FUNCTION_BLOCK FB_FileCopy
(*SwenChen 2011.4.13 ÐÞ¸ÄÓÚ°ïÖúÎÄ¼þ*)
VAR_INPUT
	srcNetId				: T_AmsNetId;	(* TwinCAT network address of the source file *)
	srcFileName			: T_MaxString;	(* source file path and name *)
	destNetId			: T_AmsNetId;	(* TwinCAT network address of the destination file *)
	destFileName		: T_MaxString;  (* destination file path and name *)
	bExecute			: BOOL;			(* rising edge start fb execution *)
	tAdsTimeOut			: TIME;			(* ads timeout *)
	cbReadLen			: UDINT;
END_VAR
VAR_OUTPUT
	bBusy				:BOOL;
	bError				:BOOL;
	nErrId				:UDINT;
END_VAR
VAR
	fbFileOpen			:FB_FileOpen;
	fbFileClose			:FB_FileClose;
	fbFileRead			:FB_FileRead;
	fbFileWrite			:FB_FileWrite;

	hSrcFile				:UINT	:= 0;(* file handle of the source file *)
	hDestFile			:UINT	:= 0;(* file handle of the destination file *)

	Step				:DWORD;
	RisingEdge			:R_TRIG;

	buffRead				:ARRAY[1..30000] OF BYTE;(* buffer *)
	cbReadLength		:UDINT:=0;
	TimeCount			:INT;
END_VAR

RisingEdge(CLK:=bExecute);
IF RisingEdge.Q THEN
	IF NOT bBusy THEN
		bBusy := TRUE;
		bError:= FALSE;
		nErrId:=0;
		Step := 1;
		cbReadLength:=0;
		hSrcFile:=0;
		hDestFile:=0;
		TimeCount:=0;
	END_IF
END_IF

IF bBusy THEN
	TimeCount:=TimeCount+1;
END_IF


CASE Step OF
	0:	(* do nothing *)
		;

	1:	(* open source file *)
		fbFileOpen(  bExecute := FALSE  );
		fbFileOpen( 	sNetId := srcNetId,
						sPathName := srcFileName,
						nMode := FOPEN_MODEREAD OR FOPEN_MODEBINARY(*FOPEN_MODETEXT*),
						ePath := PATH_GENERIC,
						tTimeout := tAdsTimeout,
						bExecute := TRUE );
		Step := Step + 1;

	2:
		fbFileOpen( bExecute := FALSE );
		IF ( NOT fbFileOpen.bBusy ) THEN
			IF ( fbFileOpen.bError ) THEN
				nErrId := fbFileOpen.nErrId;
				bError := TRUE;
				Step := 50;
			ELSE
				hSrcFile := fbFileOpen.hFile;
				Step := Step + 1;
			END_IF
		END_IF

	3:	(* open destination file *)
		fbFileOpen(  bExecute := FALSE  );
		fbFileOpen( 	sNetId := destNetId,
						sPathName := destFileName,
						nMode := FOPEN_MODEWRITE OR FOPEN_MODEBINARY(*FOPEN_MODETEXT*),
						ePath := PATH_GENERIC,
						tTimeout := tAdsTimeout,
						bExecute := TRUE );
		Step := Step+1;

	4:
		fbFileOpen(  bExecute := FALSE  );
		IF ( NOT fbFileOpen.bBusy ) THEN
			IF ( fbFileOpen.bError ) THEN
				nErrId := fbFileOpen.nErrId;
				bError := TRUE;
				Step := 50;
			ELSE
				hDestFile := fbFileOpen.hFile;
				Step := Step + 1;
			END_IF
		END_IF

	5:	(*read data from source file*)
		cbReadLength := 0;
		fbFileRead( bExecute:= FALSE );
		fbFileRead( 	sNetId:=SrcNetId,
						hFile:=hSrcFile,
						pReadBuff:= ADR(buffRead),
						cbReadLen:= (*SIZEOF(buffRead)*)cbReadLen,
						bExecute:=TRUE,
						tTimeout:=tAdsTimeOut );
		Step := Step + 1;

	6:
		fbFileRead( bExecute:= FALSE );
		IF ( NOT fbFileRead.bBusy ) THEN
			IF ( fbFileRead.bError ) THEN
				nErrId := fbFileRead.nErrId;
				bError := TRUE;
				Step := 50;
			ELSE
				cbReadLength := fbFileRead.cbRead;
				Step := Step + 1;
			END_IF
		END_IF

	7:	(*write data to destination file*)
		fbFileWrite( bExecute := FALSE );
		fbFileWrite(	sNetId:=DestNetId,
						hFile:=hDestFile,
						pWriteBuff:= ADR(buffRead),
						cbWriteLen:= cbReadLength,
						bExecute:=TRUE,
						tTimeout:=tAdsTimeOut );
		Step := Step + 1;

	8:
		fbFileWrite( bExecute := FALSE );
		IF ( NOT fbFileWrite.bBusy ) THEN
			IF ( fbFileWrite.bError ) THEN
				nErrId := fbFileWrite.nErrId;
				bError := TRUE;
				Step := 50;
			ELSE
				IF fbFileRead.bEOF THEN (*Check if the EOF flag ist set *)
					Step := 50;		(*cleanup: close the destination and source files *)
				ELSE
					Step := 5; (* repeat reading *)
				END_IF
			END_IF
		END_IF

	30:	(* close the destination file *)
		fbFileClose( bExecute := FALSE );
		fbFileClose( 	sNetId:=destNetId,
						hFile:=hDestFile,
						bExecute:=TRUE,
						tTimeout:=tAdsTimeOut );
		Step := Step + 1;

	31:
		fbFileClose( bExecute := FALSE );
		IF ( NOT fbFileClose.bBusy ) THEN
			IF ( fbFileClose.bError ) THEN
				nErrId := fbFileClose.nErrId;
				bError := TRUE;
			END_IF
			Step := 50;
			hDestFile := 0;
		END_IF

	40: (* close source file *)
		fbFileClose( bExecute := FALSE );
		fbFileClose( 	sNetId:=srcNetId,
						hFile:=hSrcFile,
						bExecute:=TRUE,
						tTimeout:=tAdsTimeOut );
		Step := Step + 1;

	41:
		fbFileClose( bExecute := FALSE );
		IF ( NOT fbFileClose.bBusy ) THEN
			IF ( fbFileClose.bError ) THEN
				nErrId := fbFileClose.nErrId;
				bError := TRUE;
			END_IF
			Step := 50;
			hSrcFile := 0;
		END_IF

	50: (*error or ready => cleanup*)
		IF ( hDestFile <> 0 ) THEN
			Step := 30; (* close the destination file*)
		ELSIF (hSrcFile <> 0 ) THEN
			Step := 40; (* close the source file *)
		ELSE
			Step := 0;	(* ready *)
			bBusy := FALSE;
		END_IF

END_CASE

END_FUNCTION_BLOCK
